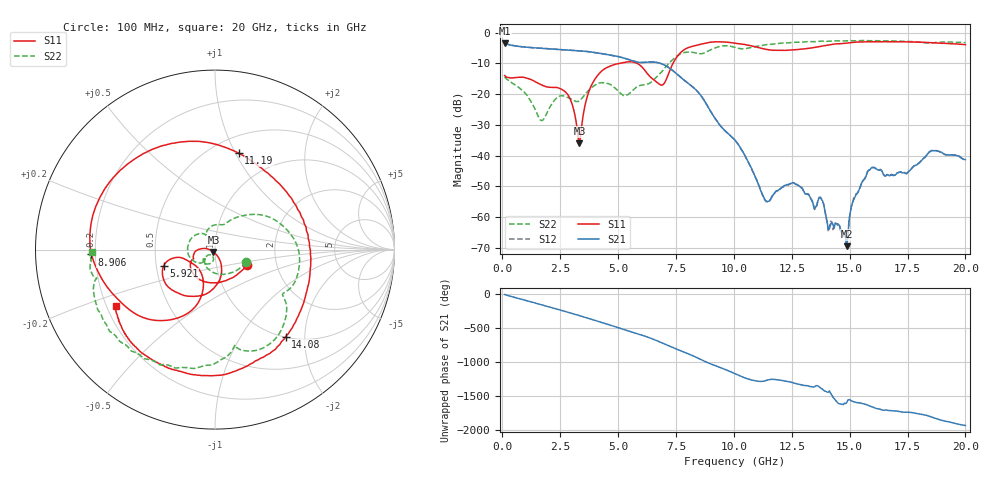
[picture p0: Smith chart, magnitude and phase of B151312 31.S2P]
!  2-Port S-parameters saved by WinCal
! VAR MeasName=S-Parameters (CALIBRATED_DATA) read from VNA (N5244A)
! VAR MeasDate=12/8/2015 5:45:52 PM
! VAR NAME=B151312 31
! VAR FILENAME=B151312 31.S2P
! VAR DATE=12/8/2015 5:45:52 PM
! VAR PHYS_PORTS=1,2
# Hz S DB R 50
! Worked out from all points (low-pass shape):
!   401 points, 100 MHz to 20 GHz, reference 50 ohm
!   highest |S21| = -3.54 dB at 100 MHz (marker M1); lowest = -69.4 dB at 14.88 GHz (marker M2)
!   |S21| within 3 dB of the highest: start of sweep to 4.022 GHz
!   lowest |S11| = -36.0 dB at 3.334 GHz (marker M3), VSWR 1.03, Z = 49.1 - j1.31 ohm
!   |S11| at or under -10 dB: start of sweep to 5.098 GHz; 5.816 GHz to 7.373 GHz (1.557 GHz wide, 23.6 % of centre)
!   |S22| runs from -28.6 to -2.6 dB; largest |S21 - S12| = 0.0013
!   S11 on the Smith chart (normalised r, x): 100 MHz: 1.41, -0.25; 5.921 GHz: 0.55, -0.11; 8.906 GHz: 0.18, -0.02; 11.19 GHz: 0.67, +1.03; 14.08 GHz: 1.01, -1.61; 20 GHz: 0.24, -0.25
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1e8  -13.99 -25.4  -3.54 -12.8  -3.54 -12.8  -14.45 -22.2
9.4575e8  -14.60 -124.2  -4.72 -93.3  -4.72 -93.3  -19.36 -116.9
1.7915e9  -17.34 -156.4  -5.15 -172.6  -5.16 -172.6  -28.07 -110.4
2.7865e9  -19.80 -177.4  -5.68 91.5  -5.68 91.5  -21.03 -137.0
3.33375e9  -35.98 -123.0  -5.94 36.8  -5.94 36.8  -22.17 -135.5
3.43325e9  -30.14 -73.4  -6.00 26.6  -6.00 26.6  -21.42 -134.2
3.83125e9  -17.48 -74.2  -6.32 -14.8  -6.32 -14.8  -18.13 -144.4
4.52775e9  -11.36 -107.9  -7.16 -88.3  -7.16 -88.3  -16.54 161.8
5.22425e9  -9.80 -133.8  -8.26 -164.7  -8.23 -164.8  -20.46 121.7
5.92075e9  -10.46 -162.5  -9.73 121.1  -9.71 120.9  -17.28 91.8
6.7665e9  -16.70 -147.2  -9.89 14.9  -9.89 14.9  -13.71 58.0
7.81125e9  -5.81 -129.6  -15.26 -134.0  -15.22 -134.3  -6.61 -1.5
8.90575e9  -3.24 -177.8  -24.45 59.8  -24.43 59.4  -5.97 -37.8
1.005e10  -3.42 131.3  -34.98 -97.7  -35.02 -98.0  -4.83 -76.0
1.119425e10  -5.15 76.1  -51.93 149.2  -51.97 150.3  -4.23 -86.9
1.338325e10  -4.98 -25.8  -54.72 70.4  -54.68 70.0  -2.99 -117.7
1.407975e10  -4.09 -50.9  -63.97 -7.6  -64.75 -2.4  -2.83 -126.4
1.487575e10  -3.44 -74.4  -69.44 -162.4  -69.14 -157.7  -2.69 -135.2
1.5821e10  -3.02 -98.1  -44.80 153.7  -44.70 153.1  -2.65 -144.9
1.67165e10  -3.01 -113.9  -46.57 80.7  -46.34 80.8  -2.69 -153.0
1.855725e10  -3.31 -138.0  -38.40 -18.4  -38.32 -18.6  -3.37 -166.5
2e10  -3.95 -150.5  -41.32 -138.9  -41.23 -140.3  -3.26 -178.8
